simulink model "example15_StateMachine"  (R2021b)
settings: Solver=FixedStepAuto  StartTime=0  StopTime=inf  FixedStep=0.5  RelTol=1e-3  EnableMultiTasking=on
undefined symbols (not defined in the file or in its folder): based, case, classic, default, dsPic33, MCC, Microchip, PIC24
libraries: embeddedCreatorLib x19, emMBSlaveLib x1

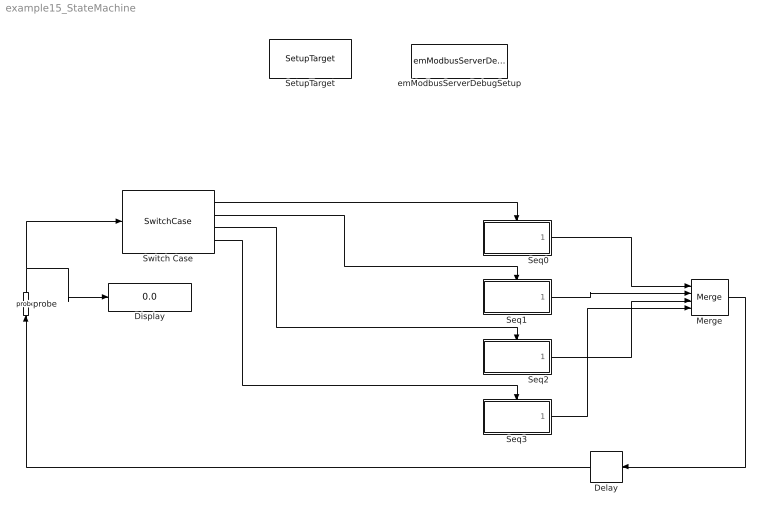
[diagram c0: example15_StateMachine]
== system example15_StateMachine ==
  Delay : Delay  DelayLength=1  InitialCondition=0
  Display : Display
  Merge : Merge  Inputs=4
  Seq0 : Subsystem  Tag=MyState  TreatAsAtomicUnit=on
  Seq1 : Subsystem  Tag=MyState  TreatAsAtomicUnit=on
  Seq2 : Subsystem  Tag=MyState  TreatAsAtomicUnit=on
  Seq3 : Subsystem  Tag=MyState  TreatAsAtomicUnit=on
  SetupTarget : embeddedCreatorLib/SetupTarget  Tag=SetupTarget  Priority=0  c_platform=Microchip PIC24/dsPic33 based on MCC classic  c_debug=on
  Switch Case : SwitchCase  CaseConditions={0, 1, 2}
  emModbusServerDebugSetup : emMBSlaveLib/emModbusServerDebugSetup  Tag=emModbusSlaveSetup  c_objID=0  c_uartNo=2  c_baudrate=19200  c_serverID=1  c_baudrate4PC=19200  c_forceLongerSpace=on  c_holdingRegsQTY=0  c_minHoldingAddr=789  c_inputRegsQTY=0  c_minInputRegAddr=20  c_coilRegsQTY=0  c_minCoilAddr=30  c_discreteRegsQTY=0  c_minDiscreteAddr=40  c_enableDebug=on  c_breakpointMaxQTY=0  c_probeMaxWordQTY=100  c_emWaitQTY=3  g_COMPortNo=COM5  c_Name_method=By physical port name and bit number  c_PortName=B  c_BitNo=11  c_TxEnable485="\"LATBbits.LATB11\""  c_TxEnable485Polarity=on
  probe : embeddedCreatorLib/probe  Tag=emProbe  c_ObjID=0  c_serverID=1  c_UartNo=2  c_StartAddr=5  c_ConstantDataSource=off
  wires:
  Switch Case/1 -> Seq0/Action
  Switch Case/2 -> Seq1/Action
  Seq0/1(Out1) -> Merge/1
  Seq1/1(Out1) -> Merge/2
  Merge/1 -> Delay/1
  Delay/1 -> probe/1
  probe/1 -> Display/1, Switch Case/1
  Switch Case/3 -> Seq2/Action
  Seq2/1(Out1) -> Merge/3
  Switch Case/4 -> Seq3/Action
  Seq3/1(Out1) -> Merge/4

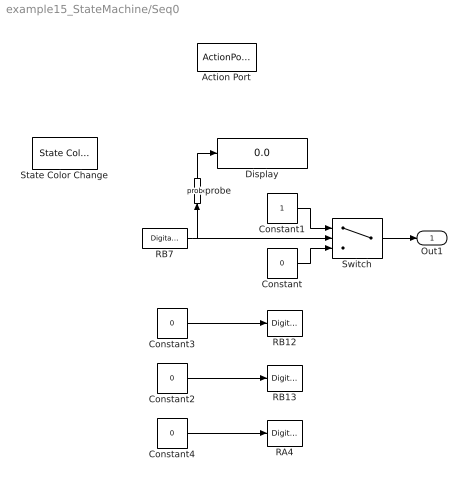
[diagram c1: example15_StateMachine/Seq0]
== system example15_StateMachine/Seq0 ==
  Action Port : ActionPort  ActionPortLabel=case [ 0 ]:
  Constant : Constant  Value=0  OutDataTypeStr=uint8
  Constant1 : Constant  OutDataTypeStr=uint8
  Constant2 : Constant  Value=0  OutDataTypeStr=boolean
  Constant3 : Constant  Value=0  OutDataTypeStr=boolean
  Constant4 : Constant  Value=0  OutDataTypeStr=boolean
  Display : Display
  RA4 : embeddedCreatorLib/Digital Output  c_Name_method=By physical port name and bit number  c_PortName=A  c_BitNo=4  c_DinAccessName="\"LATAbits.LATA4\""  c_initialV=1  c_sampleTime=-1
  RB12 : embeddedCreatorLib/Digital Output  c_Name_method=By physical port name and bit number  c_PortName=B  c_BitNo=12  c_DinAccessName="\"LATBbits.LATB12\""  c_initialV=1  c_sampleTime=-1
  RB13 : embeddedCreatorLib/Digital Output  c_Name_method=By physical port name and bit number  c_PortName=B  c_BitNo=13  c_DinAccessName="\"LATBbits.LATB13\""  c_initialV=1  c_sampleTime=-1
  RB7 : embeddedCreatorLib/Digital Input  c_Name_method=By physical port name and bit number  c_PortName=B  c_BitNo=7  c_DinAccessName="\"PORTBbits.RB7\""  c_EnableFilter=on  c_Filter_method=Continuous sample multiple times in one sample period  c_filterQTY=12  c_initialV=0  c_sampleTime=-1
  State Color Change : embeddedCreatorLib/State Color Change  g_tag="\"MyState\""  g_QTY=4
  Switch : Switch  Criteria=u2 > Threshold
  probe : embeddedCreatorLib/probe  Tag=emProbe  c_ObjID=1  c_serverID=1  c_UartNo=2  c_StartAddr=6  c_ConstantDataSource=off
  Out1 : Outport
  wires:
  Constant/1 -> Switch/3
  Constant1/1 -> Switch/1
  Switch/1 -> Out1/1
  RB7/1 -> probe/1, Switch/2
  Constant3/1 -> RB12/1
  probe/1 -> Display/1
  Constant2/1 -> RB13/1
  Constant4/1 -> RA4/1

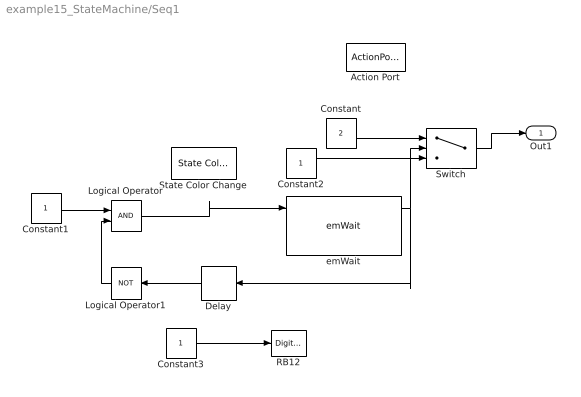
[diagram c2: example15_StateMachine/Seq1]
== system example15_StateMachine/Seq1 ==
  Action Port : ActionPort  ActionPortLabel=case [ 1 ]:
  Constant : Constant  Value=2  OutDataTypeStr=uint8
  Constant1 : Constant  OutDataTypeStr=boolean
  Constant2 : Constant  OutDataTypeStr=uint8
  Constant3 : Constant  OutDataTypeStr=boolean
  Delay : Delay  DelayLength=1
  Logical Operator : Logic  AllPortsSameDT=off  OutDataTypeStr=boolean
  Logical Operator1 : Logic  Operator=NOT  AllPortsSameDT=off  OutDataTypeStr=boolean
  RB12 : embeddedCreatorLib/Digital Output  c_Name_method=By physical port name and bit number  c_PortName=B  c_BitNo=12  c_DinAccessName="\"LATBbits.LATB12\""  c_initialV=1  c_sampleTime=-1
  State Color Change : embeddedCreatorLib/State Color Change  g_tag="\"MyState\""  g_QTY=4
  Switch : Switch  Criteria=u2 > Threshold
  emWait : embeddedCreatorLib/emWait  Tag=emWait  c_hours=0  c_minutes=0  c_seconds=12  c_ms=0  c_ObjID=0  c_serverID=1  c_UartNo=2  c_sampleTime=-1
  Out1 : Outport
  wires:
  Constant1/1 -> Logical Operator/1
  Logical Operator/1 -> emWait/1
  Logical Operator1/1 -> Logical Operator/2
  Constant/1 -> Switch/1
  Switch/1 -> Out1/1
  Constant2/1 -> Switch/3
  emWait/1 -> Delay/1, Switch/2
  Delay/1 -> Logical Operator1/1
  Constant3/1 -> RB12/1

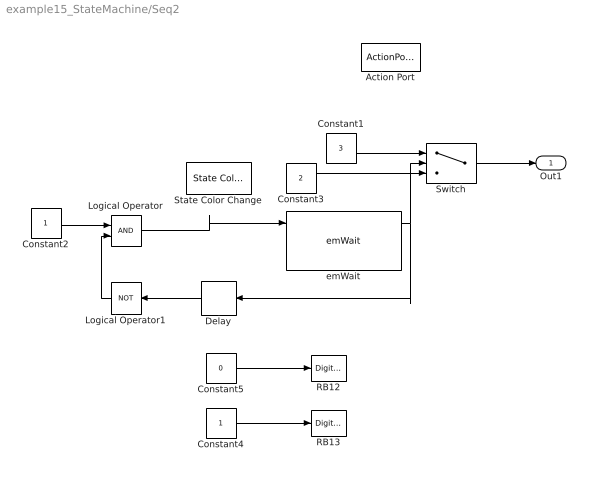
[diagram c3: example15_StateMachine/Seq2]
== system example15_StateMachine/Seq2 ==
  Action Port : ActionPort  ActionPortLabel=case [ 2 ]:
  Constant1 : Constant  Value=3  OutDataTypeStr=uint8
  Constant2 : Constant  OutDataTypeStr=boolean
  Constant3 : Constant  Value=2  OutDataTypeStr=uint8
  Constant4 : Constant  OutDataTypeStr=boolean
  Constant5 : Constant  Value=0  OutDataTypeStr=boolean
  Delay : Delay  DelayLength=1
  Logical Operator : Logic  AllPortsSameDT=off  OutDataTypeStr=boolean
  Logical Operator1 : Logic  Operator=NOT  AllPortsSameDT=off  OutDataTypeStr=boolean
  RB12 : embeddedCreatorLib/Digital Output  c_Name_method=By physical port name and bit number  c_PortName=B  c_BitNo=12  c_DinAccessName="\"LATBbits.LATB12\""  c_initialV=1  c_sampleTime=-1
  RB13 : embeddedCreatorLib/Digital Output  c_Name_method=By physical port name and bit number  c_PortName=B  c_BitNo=13  c_DinAccessName="\"LATBbits.LATB13\""  c_initialV=1  c_sampleTime=-1
  State Color Change : embeddedCreatorLib/State Color Change  g_tag="\"MyState\""  g_QTY=4
  Switch : Switch  Criteria=u2 > Threshold
  emWait : embeddedCreatorLib/emWait  Tag=emWait  c_hours=0  c_minutes=0  c_seconds=12  c_ms=0  c_ObjID=1  c_serverID=1  c_UartNo=2  c_sampleTime=-1
  Out1 : Outport
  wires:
  Logical Operator1/1 -> Logical Operator/2
  Logical Operator/1 -> emWait/1
  Delay/1 -> Logical Operator1/1
  Constant1/1 -> Switch/1
  Constant2/1 -> Logical Operator/1
  Constant3/1 -> Switch/3
  emWait/1 -> Delay/1, Switch/2
  Switch/1 -> Out1/1
  Constant4/1 -> RB13/1
  Constant5/1 -> RB12/1

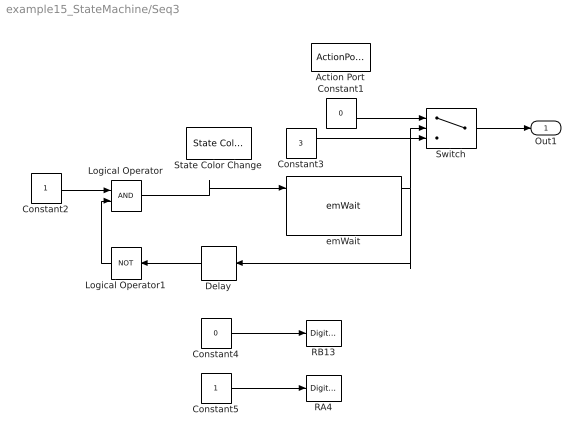
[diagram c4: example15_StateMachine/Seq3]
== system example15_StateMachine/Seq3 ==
  Action Port : ActionPort  ActionPortLabel=default:
  Constant1 : Constant  Value=0  OutDataTypeStr=uint8
  Constant2 : Constant  OutDataTypeStr=boolean
  Constant3 : Constant  Value=3  OutDataTypeStr=uint8
  Constant4 : Constant  Value=0  OutDataTypeStr=boolean
  Constant5 : Constant  OutDataTypeStr=boolean
  Delay : Delay  DelayLength=1
  Logical Operator : Logic  AllPortsSameDT=off  OutDataTypeStr=boolean
  Logical Operator1 : Logic  Operator=NOT  AllPortsSameDT=off  OutDataTypeStr=boolean
  RA4 : embeddedCreatorLib/Digital Output  c_Name_method=By physical port name and bit number  c_PortName=A  c_BitNo=4  c_DinAccessName="\"LATAbits.LATA4\""  c_initialV=1  c_sampleTime=-1
  RB13 : embeddedCreatorLib/Digital Output  c_Name_method=By physical port name and bit number  c_PortName=B  c_BitNo=13  c_DinAccessName="\"LATBbits.LATB13\""  c_initialV=1  c_sampleTime=-1
  State Color Change : embeddedCreatorLib/State Color Change  g_tag="\"MyState\""  g_QTY=4
  Switch : Switch  Criteria=u2 > Threshold
  emWait : embeddedCreatorLib/emWait  Tag=emWait  c_hours=0  c_minutes=0  c_seconds=12  c_ms=0  c_ObjID=2  c_serverID=1  c_UartNo=2  c_sampleTime=-1
  Out1 : Outport
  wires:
  Constant3/1 -> Switch/3
  Switch/1 -> Out1/1
  Constant2/1 -> Logical Operator/1
  Constant1/1 -> Switch/1
  Logical Operator/1 -> emWait/1
  emWait/1 -> Delay/1, Switch/2
  Logical Operator1/1 -> Logical Operator/2
  Delay/1 -> Logical Operator1/1
  Constant5/1 -> RA4/1
  Constant4/1 -> RB13/1
